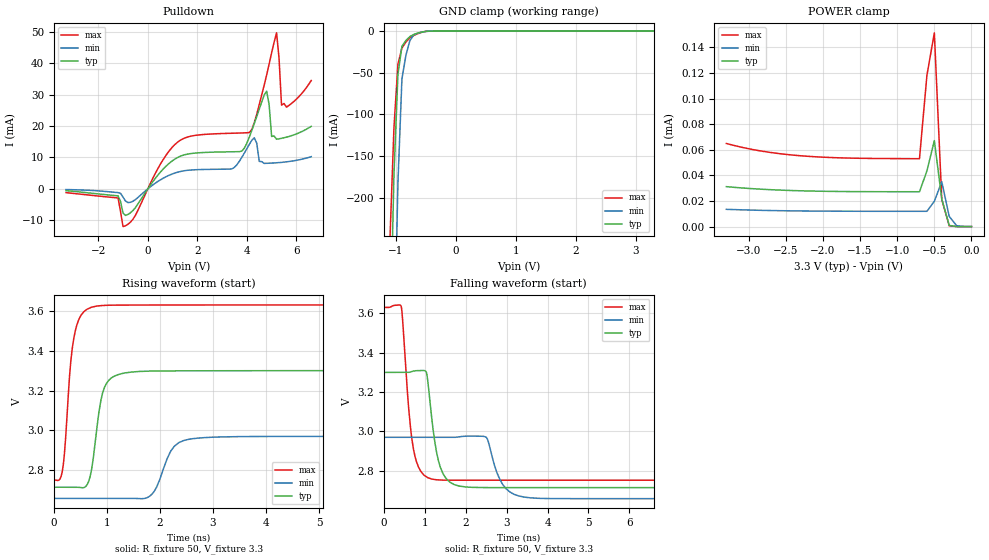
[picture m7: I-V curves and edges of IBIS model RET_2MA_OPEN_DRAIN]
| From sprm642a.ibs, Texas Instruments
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|   Model Cell RET_2MA_OPEN_DRAIN
|RET_2MA_OPEN_DRAIN
[Model]   RET_2MA_OPEN_DRAIN
Model_type   I/O_open_drain
Polarity   Inverting
Enable   Active-Low
Vinl =  0.8
Vinh =  2
Cref =  15.0000pF
Rref =  100.0000M
Vref =  0V
Vmeas =  1.65
C_comp   5.345208p   4.561426p   6.022817p
[Model Spec]
Vinl   0.8   0.8   0.8
Vinh   2   2   2
[Temperature Range]   25   155   -40
[Voltage Range]   3.3   2.97   3.63
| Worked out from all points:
|   slope of the pulldown table from 0 to 0.495 V, typ, clamps not added: 95.1 ohm
|   GND clamp passes 1 mA (typ) near -0.55 V on its own axis
|   rising waveform, R_fixture 50, V_fixture 3.3: 20-80 % time 187ps typ, 291ps min, 158ps max; typ from 2.71 V to 3.3 V
|   falling waveform, R_fixture 50, V_fixture 3.3: 20-80 % time 250ps typ, 339ps min, 215ps max; typ from 3.3 V to 2.71 V
| Nom Voltages:
|   BIASFET=3.3, VDD=1.2, VDDS=3.3, VSS=0
| Min Voltages:
|   BIASFET=2.97, VDD=1.08, VDDS=2.97, VSS=0
| Max Voltages:
|   BIASFET=3.63, VDD=1.32, VDDS=3.63, VSS=0
[POWER_clamp]
|   voltage   I(typ)   I(min)   I(max)
-3.3V     31.22uA    13.5uA     64.95uA
-2.8V     29.13uA    12.67uA    58.77uA
-2.3V     27.98uA    12.22uA    55.36uA
-1.7V     27.4uA     12.01uA    53.62uA
-700mV    27.24uA    11.95uA    53.12uA
-600mV    43.52uA    11.94uA    118.2uA
-500mV    67.2uA     19.79uA    151.5uA
-400mV    21.58uA    35.09uA    21.1uA
-300mV    927.4nA    7.958uA    611.4nA
-200mV    28.93nA    716.3nA    11.51nA
0V        697pA      39.48nA    568.3pA
[Pulldown]
|   voltage   I(typ)   I(min)   I(max)
-3.3V     -580.7uA   -221.2uA   -1.206mA
-1.2V     -2.224mA   -1.185mA   -2.903mA
-1V       -7.701mA   -2.63mA    -12.01mA
1.2V      9.981mA    5.309mA    14.86mA
3.4V      11.82mA    6.395mA    17.72mA
4.1V      16.51mA    14.18mA    17.95mA
4.3V      20.83mA    16.28mA    21.06mA
4.8V      31.11mA    8.148mA    36.31mA
5V        16.71mA    8.219mA    43.35mA
5.2V      15.82mA    8.317mA    49.72mA
5.4V      16.11mA    8.446mA    26.68mA
6.6V      19.93mA    10.26mA    34.53mA
[GND_clamp]
|   voltage   I(typ)   I(min)   I(max)
-3.3V     -16.36A    -15.08A    -17.18A
-1.1V     -382.1mA   -717.8mA   -250.1mA
-1.033V   -173.3mA   -402.2mA   -116.4mA
-966.7mV  -52.02mA   -182.1mA   -39.81mA
-900mV    -18.21mA   -57.43mA   -20.34mA
-833.3mV  -11.36mA   -28.88mA   -13.17mA
-766.7mV  -6.618mA   -11.27mA   -8.134mA
-700mV    -3.983mA   -4.59mA    -5.247mA
-500mV    -328.3uA   -481.4uA   -374.5uA
-366.7mV  -15.94uA   -50.74uA   -14.83uA
3.3V      697pA      15.84uA    426.1pA
[Ramp]
| variable   typ   min   max
dV/dt_f 0.35734831/0.25101078n 0.19080903/0.34043716n 0.53450667/0.21602902n
dV/dt_r 0.51636145/0.48463515n 0.31304585/0.84202478n 0.71397486/0.35777031n
R_load = 50
[Rising Waveform]
R_fixture = 50
V_fixture = 3.3
V_fixture_min = 2.97
V_fixture_max = 3.63
|   time   V(typ)   V(min)   V(max)
0s        2.714V     2.658V     2.751V
178.3ps   2.714V     2.658V     2.827V
399.7ps   2.715V     2.658V     3.495V
653.4ps   2.741V     2.658V     3.612V
795.2ps   2.974V     2.658V     3.624V
992.8ps   3.236V     2.658V     3.628V
1.593ns   3.296V     2.657V     3.629V
2.273ns   3.299V     2.921V     3.63V
2.829ns   3.299V     2.963V     3.63V
20.01ns   3.3V       2.97V      3.63V
[Falling Waveform]
R_fixture = 50
V_fixture = 3.3
V_fixture_min = 2.97
V_fixture_max = 3.63
|   time   V(typ)   V(min)   V(max)
0s        3.3V       2.97V      3.63V
420.4ps   3.3V       2.97V      3.636V
713.3ps   3.306V     2.97V      2.918V
1.038ns   3.3V       2.97V      2.769V
1.164ns   3.075V     2.97V      2.758V
1.436ns   2.789V     2.97V      2.752V
1.984ns   2.718V     2.976V     2.752V
2.508ns   2.715V     2.969V     2.752V
3.572ns   2.714V     2.663V     2.752V
20.01ns   2.714V     2.658V     2.752V
